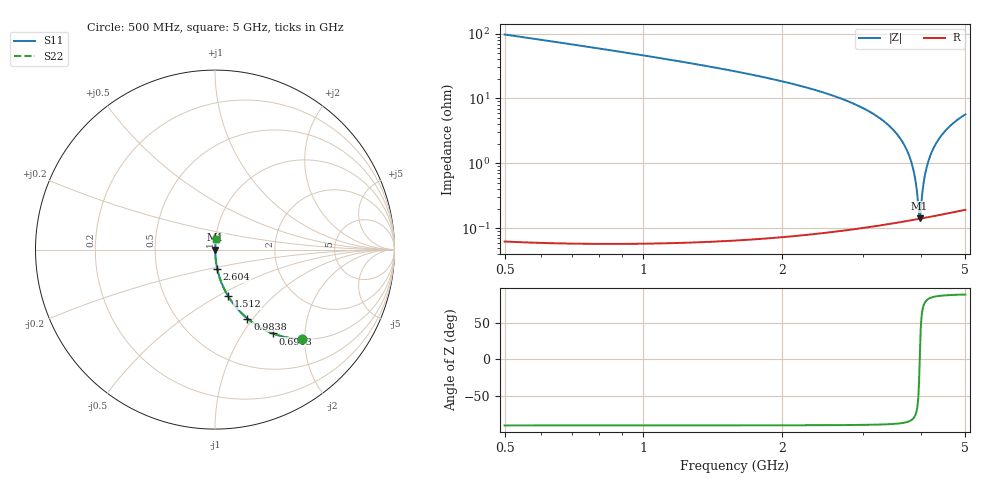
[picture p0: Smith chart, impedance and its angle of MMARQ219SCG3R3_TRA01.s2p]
! MMARQ219SCG3R3_TRA01  S-PARAMETER MODEL  ( General Type )
! Model Generated by TAIYO YUDEN Corporation (http://www.ty-top.com)
! Version 1.0
! TAIYO YUDEN Control No. 160201
! Copyright(c) 2016 TAIYO YUDEN CO.,LTD. All Rights Reserved.
! Product Description (link to TY-COMPAS)
! https://ds.yuden.co.jp/TYCOMPAS/or/detail?pn=MMARQ219SCG3R3BTRA01&u=M
! Products Name : Multilayer Ceramic Capacitors
! Characteristics :
!  Capacitance : 3.3 pF , Rated Voltage : 250V , TCC : CG / C0G
!  Case Size : 2.0 x 1.25 / 0.079 x 0.049 [mm/inch] , Thickness : 0.85 / 0.033 [mm/inch]
!  (Conditions: Temperature = 25 degC , DC Bias Current/Voltage = 0A / 0V)
! External Node Assignments :
!  1  o---| |---o  2
! GND o---------o GND
! Frequency Range : 500MHz  -  5000MHz  [ 401 STEP ]
# MHz S RI R 50
! Freq[MHz].  S11 Real  S11 Imag  S21 Real  S21 Imag  S12 Real  S12 Imag  S22 Real  S22 Imag
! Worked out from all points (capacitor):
!   401 points, 500 MHz to 5 GHz, reference 50 ohm
!   read as one part in series: C = 3.24 pF near 522.5 MHz
!   lowest |Z| = 142 mohm at 3.976 GHz (marker M1)
!   series resonance near 3.98 GHz, so ESL is about 490 pH
!   S11 on the Smith chart (normalised r, x): 500 MHz: 1.00, -1.94; 691.2 MHz: 1.00, -1.38; 983.8 MHz: 1.00, -0.94; 1.512 GHz: 1.00, -0.56; 2.604 GHz: 1.00, -0.22; 5 GHz: 1.00, +0.11
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500  0.4839 -0.4994  0.5161 0.4994  0.5161 0.4994  0.4839 -0.4994
691.25  0.3227 -0.4671  0.6773 0.4671  0.6773 0.4671  0.3227 -0.4671
983.75  0.1809 -0.3843  0.8191 0.3843  0.8191 0.3843  0.1809 -0.3843
1253.75  0.1114 -0.3138  0.8886 0.3138  0.8886 0.3138  0.1114 -0.3138
1512.5  0.0723 -0.2579  0.9277 0.2579  0.9277 0.2579  0.0723 -0.2579
2007.5  0.0329 -0.1765  0.9671 0.1765  0.9671 0.1765  0.0329 -0.1765
2603.75  0.0124 -0.1066  0.9876 0.1066  0.9876 0.1066  0.0124 -0.1066
2750  0.00956 -0.0925  0.9904 0.0925  0.9904 0.0925  0.00956 -0.0925
3188.75  0.00411 -0.0549  0.9959 0.0549  0.9959 0.0549  0.00411 -0.0549
3503.75  0.00219 -0.0315  0.9978 0.0315  0.9978 0.0315  0.00219 -0.0315
3683.75  0.00163 -0.0191  0.9984 0.0191  0.9984 0.0191  0.00163 -0.0191
3818.75  0.00143 -0.0102  0.9986 0.0102  0.9986 0.0102  0.00143 -0.0102
3897.5  0.00139 -0.00515  0.9986 0.00515  0.9986 0.00515  0.00139 -0.00515
3953.75  0.00139 -0.00161  0.9986 0.00161  0.9986 0.00161  0.00139 -0.00161
3976.25  0.0014 -0.000216  0.9986 0.000216  0.9986 0.000216  0.0014 -0.000216
3998.75  0.00141 0.00117  0.9986 -0.00117  0.9986 -0.00117  0.00141 0.00117
4043.75  0.00144 0.00393  0.9986 -0.00393  0.9986 -0.00393  0.00144 0.00393
4100  0.00151 0.00734  0.9985 -0.00734  0.9985 -0.00734  0.00151 0.00734
4167.5  0.00162 0.0114  0.9984 -0.0114  0.9984 -0.0114  0.00162 0.0114
4257.5  0.00181 0.0166  0.9982 -0.0166  0.9982 -0.0166  0.00181 0.0166
4550  0.00277 0.033  0.9972 -0.033  0.9972 -0.033  0.00277 0.033
5000  0.00513 0.0565  0.9949 -0.0565  0.9949 -0.0565  0.00513 0.0565
